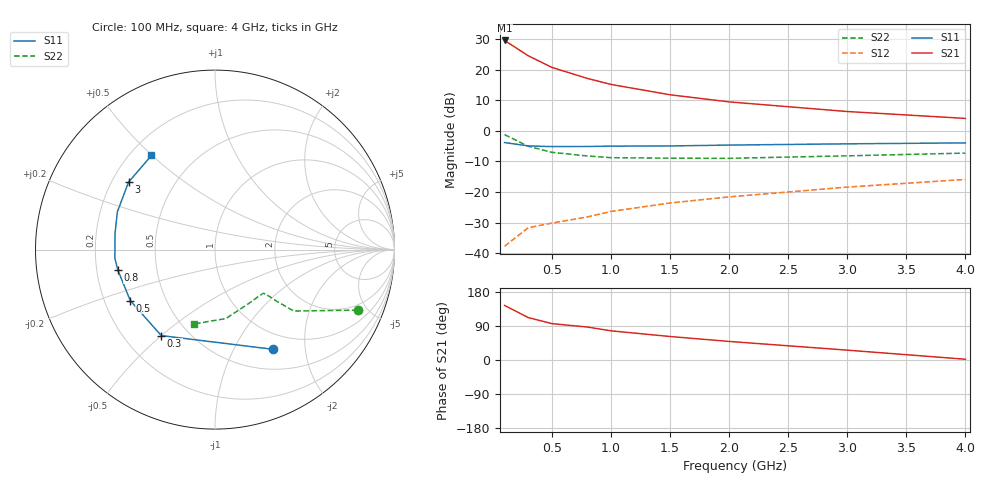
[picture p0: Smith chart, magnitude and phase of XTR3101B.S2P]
! HXTR-3101 Common Emitter
! Vce=10V  Ic=15mA
# ghz s ma r 50
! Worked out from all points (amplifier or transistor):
!   9 points, 100 MHz to 4 GHz, reference 50 ohm
!   highest |S21| = 29.5 dB at 100 MHz (marker M1)
!   |S21| within 3 dB of that: start of sweep to 219.9 MHz
!   unconditionally stable (mu >= 1): 853.1 MHz to 2.744 GHz
!   at 300 MHz: K = 0.53, MSG = 28.1 dB, |S12| = -31.7 dB
!   at 1 GHz: K = 1.03, MAG = 19.7 dB, |S12| = -26.4 dB
!   at 4 GHz: K = 0.84, MSG = 10.0 dB, |S12| = -15.9 dB
!   S11 on the Smith chart (normalised r, x): 100 MHz: 0.77, -1.44; 300 MHz: 0.35, -0.50; 500 MHz: 0.31, -0.25; 800 MHz: 0.29, -0.10; 3 GHz: 0.27, +0.32; 4 GHz: 0.28, +0.50
0.1  0.641 -60.0  29.85 144.0  0.013 57.0  0.863 -23.0
0.3  0.565 -122.0  16.78 112.0  0.026 44.0  0.556 -38.0
0.5  0.551 -149.0  10.84 96.0  0.031 44.0  0.444 -40.0
0.8  0.553 -168.0  7.16 87.0  0.039 50.0  0.387 -41.0
1  0.56 -175.0  5.71 77.0  0.048 49.0  0.363 -42.0
1.5  0.564 171.0  3.87 62.0  0.066 54.0  0.356 -47.0
2  0.583 159.0  2.96 49.0  0.083 52.0  0.354 -56.0
3  0.611 142.0  2.06 26.0  0.12 47.0  0.389 -81.0
4  0.633 124.0  1.59 2.0  0.16 39.0  0.431 -106.0
